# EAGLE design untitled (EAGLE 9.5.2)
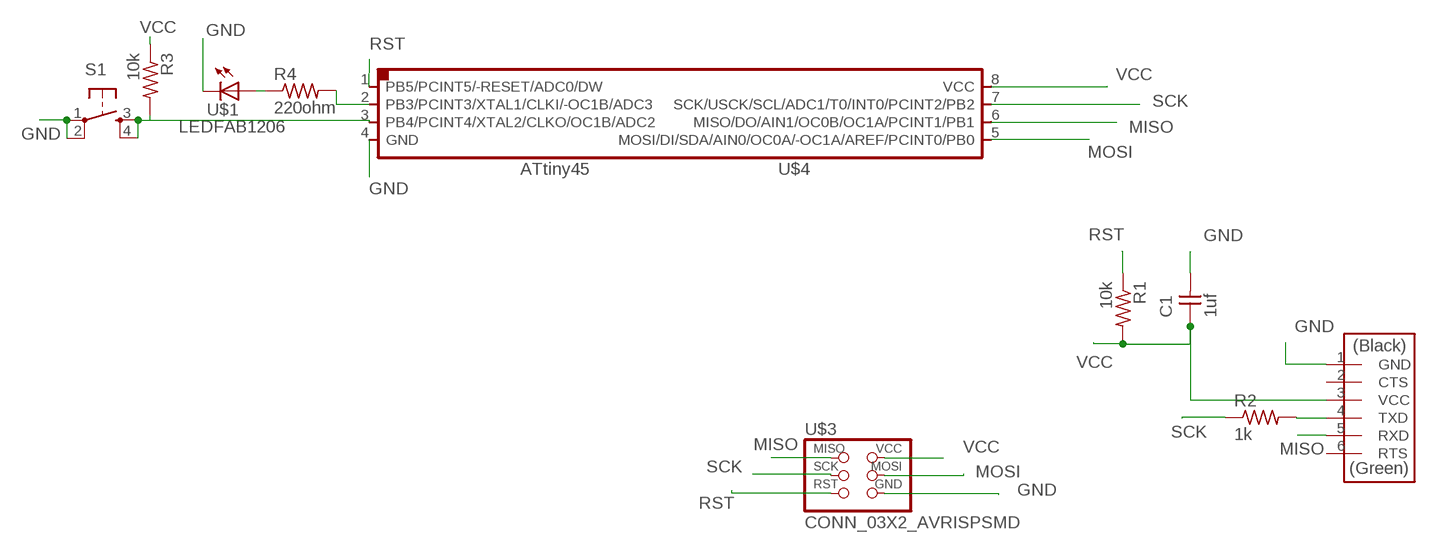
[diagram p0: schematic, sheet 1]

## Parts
C1  1uf  CAP_UNPOLARIZEDFAB  [C1206FAB]
R1  10k  R1206FAB  [R1206FAB]
R2  1k  R1206FAB  [R1206FAB]
R3  10k  R1206FAB  [R1206FAB]
R4  220ohm  R1206FAB  [R1206FAB]
S1  SW_SWITCH_TACTILE_6MM6MM_SWITCH  [6MM_SWITCH]
U$1  LEDFAB1206  [LED1206FAB]
U$2  CONN_06_FTDI-SMD-HEADER  [1X06SMD]
U$3  CONN_03X2_AVRISPSMD  [2X03SMD]
U$4  UC_ATTINY45SI  [SOIC8]

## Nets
GND: C1.2 S1.1(P) S1.2(P1) U$1.2(C) U$2.1(GND) U$3.6(GND) U$4.4(GND)
MISO: U$2.5(RXD) U$3.1(MISO) U$4.6(MISO/DO/AIN1/OC0B/OC1A/PCINT1/PB1)
MOSI: U$3.4(MOSI) U$4.5(MOSI/DI/SDA/AIN0/OC0A/-OC1A/AREF/PCINT0/PB0)
N$1: R4.2 U$4.2(PB3/PCINT3/XTAL1/CLKI/-OC1B/ADC3)
N$2: R2.2 U$2.4(TXD)
N$3: R4.1 U$1.1(A)
N$5: R3.2 S1.3(S) S1.4(S1) U$4.3(PB4/PCINT4/XTAL2/CLKO/OC1B/ADC2)
RST: R1.1 U$3.5(RST) U$4.1(PB5/PCINT5/-RESET/ADC0/DW)
SCK: R2.1 U$3.3(SCK) U$4.7(SCK/USCK/SCL/ADC1/T0/INT0/PCINT2/PB2)
VCC: C1.1 R1.2 R3.1 U$2.3(VCC) U$3.2(VCC) U$4.8(VCC)
Unconnected: U$2.2(CTS) U$2.6(RTS)

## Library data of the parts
C1 = fab:CAP_UNPOLARIZED
R1-R4 = fab:R: Resistor (US Symbol)
S1 = fab:SW_SWITCH_TACTILE_6MM: OMRON SWITCH
U$1 = fab:LED: LED
U$2 = fab:CONN_06_FTDI-SMD-HEADER
U$3 = fab:CONN_03X2_AVRISP
U$4 = fab:UC_ATTINY45

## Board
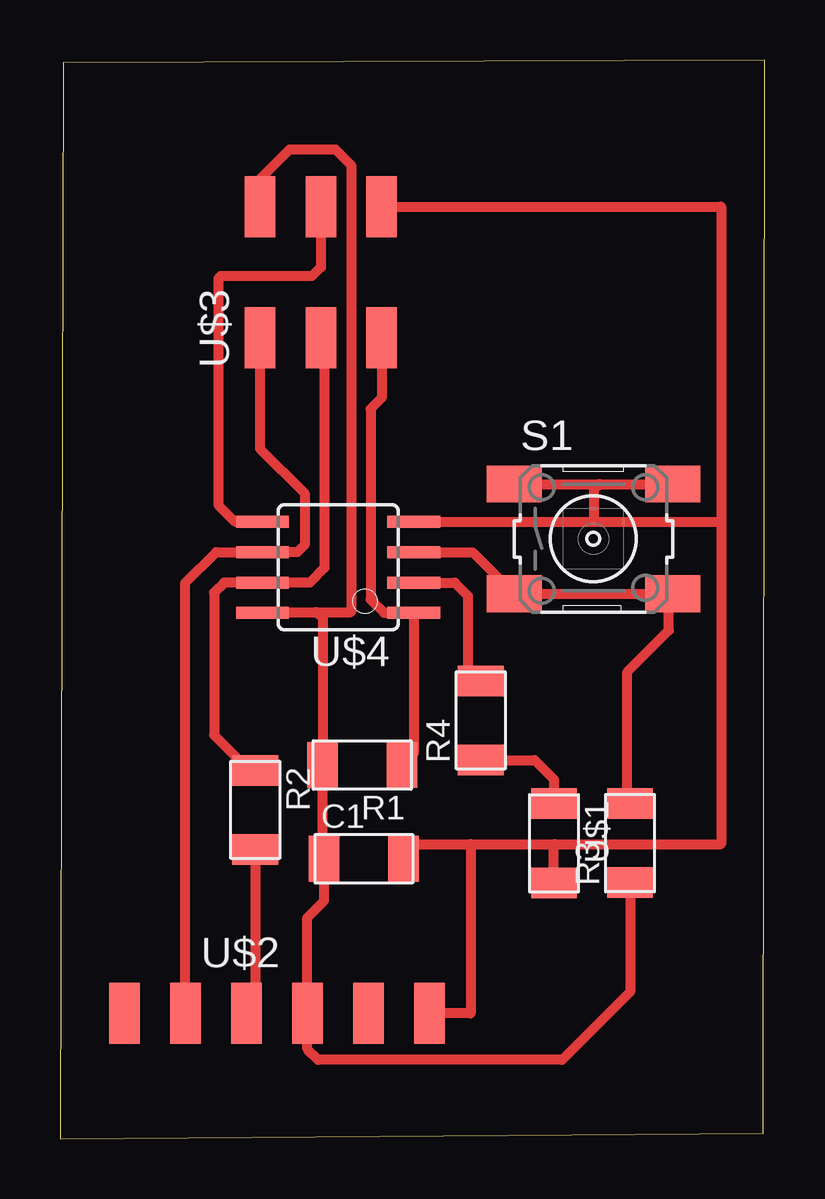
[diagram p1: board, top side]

Size 29.37 x 44.94 mm. Coordinates in mm from the lower left corner, seen from the top.
Outline: 0,0 29.31,0.22 29.37,44.94 0.13,44.83 0,0
Copper layers (1*16): Top 0.035mm / dielectric 1.5mm / Bottom 0.035mm
Design rules "default *": minimum track width 6mil, minimum drill 0.35mm, track to track 16mil, track to pad 16mil, pad to pad 16mil, via to via 16mil, smd to smd 16mil, copper to edge 40mil, drill to drill 6mil, minimum pad ring 10mil, minimum via ring 8mil, stop-mask expansion 4mil, vias tented up to drill 0mil, thermal gap 10mil

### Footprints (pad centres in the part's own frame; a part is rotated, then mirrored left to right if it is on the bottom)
C1206FAB = smd 1.27 x 1.905: 1 -1.651,0; 2 1.651,0
R1206FAB = smd 1.27 x 1.905: 1 -1.651,0; 2 1.651,0
6MM_SWITCH = smd 2.286 x 1.524: 1 -3.302,2.286; 2 3.302,2.286; 3 -3.302,-2.286; 4 3.302,-2.286
LED1206FAB = smd 1.27 x 1.905: 1 -1.651,0; 2 1.651,0
1X06SMD = smd 2.54 x 1.27: 1 0,6.35; 2 0,3.81; 3 0,1.27; 4 0,-1.27; 5 0,-3.81; 6 0,-6.35
2X03SMD = smd 2.54 x 1.27: 1 -2.54,2.54; 2 2.92,2.54; 3 -2.54,0; 4 2.92,0; 5 -2.54,-2.54; 6 2.92,-2.54
SOIC8 = smd 0.5 x 2.2: 1 -1.905,-3.154; 2 -0.645,-3.154; 3 0.625,-3.154; 4 1.895,-3.154; 5 1.905,3.154; 6 0.635,3.154; 7 -0.635,3.154; 8 -1.905,3.154

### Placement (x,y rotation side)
C1  12.66,11.66 0 top
R1  12.59,15.57 180 top
R2  8.14,13.69 270 top
R3  23.75,12.31 90 top
R4  17.53,17.42 90 top
S1  22.22,24.99 0 top
U$1  20.58,12.3 270 top
U$2  9.04,5.22 270 top
U$3  10.87,35.91 90 top
U$4  11.59,23.8 90 top

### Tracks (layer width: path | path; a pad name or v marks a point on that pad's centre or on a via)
GND
  Top 0.406: 27.55,25.7 27.55,12.27 20.61,12.27 | 17.11,12.27 17.11,5.22 U$2.1 | U$4.4 22.25,25.7 | 22.25,25.7 27.55,25.7 | U$3.6 27.55,38.83 27.55,25.7 | C1.2 14.92,12.27 17.11,12.27 | 17.11,12.27 20.61,12.27 | S1.1 22.47,27.27 | 22.47,27.27 S1.2 | 22.47,27.27 22.25,27.05 22.25,25.7 | U$1.2 20.58,12.24 20.61,12.27
MISO
  Top 0.406: U$3.1 8.33,28.74 10.19,26.88 10.19,24.74 9.89,24.44 U$4.6 6.51,24.44 5.23,23.16 U$2.5
MOSI
  Top 0.406: U$3.4 10.87,36.3 10.5,35.93 6.69,35.93 6.6,35.84 6.6,26.39 7.29,25.71 U$4.5
N$1
  Top 0.406: U$4.2 16.45,23.16 17,22.61 17,19.6 R4.2
N$2
  Top 0.406: R2.2 8.14,5.59 U$2.4
N$3
  Top 0.406: R4.1 19.77,15.77 20.58,14.96 U$1.1
N$5
  Top 0.406: U$4.3 17.19,24.43 S1.3 25.37,22.7 | 25.37,22.7 S1.4 | R3.2 23.64,14.07 23.64,19.45 25.37,21.18 25.37,22.7
RST
  Top 0.406: U$3.5 13.41,30.86 12.95,30.4 12.95,22.45 13.5,21.9 U$4.1 14.74,16.07 R1.1
SCK
  Top 0.406: U$3.3 11.02,33.22 11.02,23.77 10.41,23.17 U$4.7 6.83,23.17 6.43,22.76 6.43,16.81 7.89,15.35 R2.1
VCC
  Top 0.406: U$3.2 8.33,39.97 9.57,41.22 11.47,41.22 12.13,40.56 12.13,21.94 10.68,21.94 | U$4.8 8.48,21.94 10.68,21.94 | 10.68,21.94 10.94,21.67 R1.2 10.94,11.72 C1.1 | C1.1 | C1.1 11.01,9.91 10.31,9.21 10.31,5.37 U$2.3 10.31,3.72 10.75,3.28 20.92,3.28 23.75,6.11 R3.1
